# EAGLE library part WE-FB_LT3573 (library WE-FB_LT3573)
Flyback Converter WE-FB for LT3573 - Input voltage: 24 V - Output power: 5 W - Isolation voltage: 1.5 kV - designd for LT3573 -- Industrial input voltage
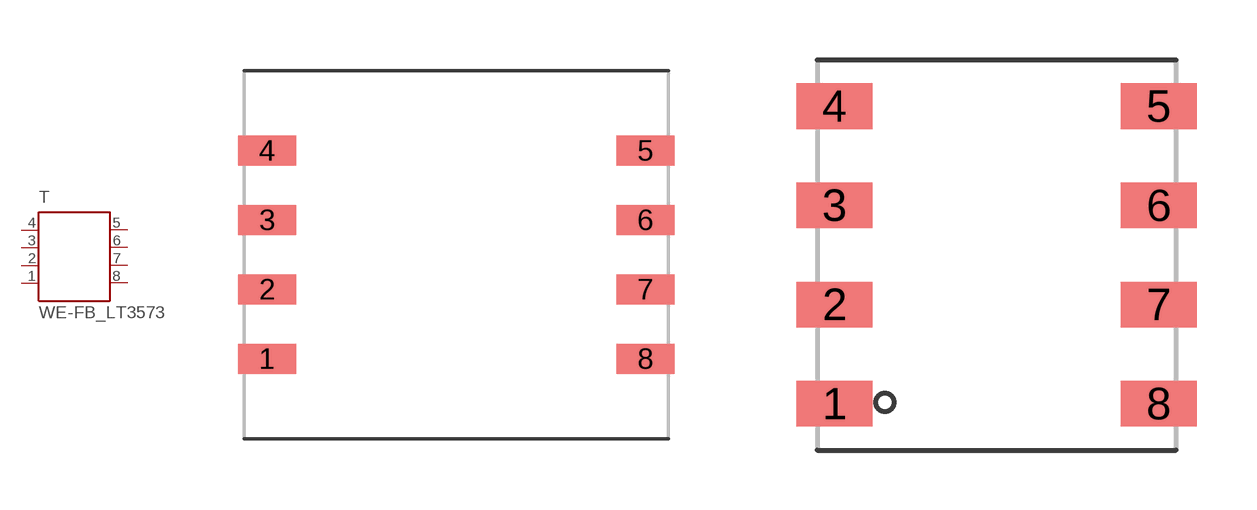
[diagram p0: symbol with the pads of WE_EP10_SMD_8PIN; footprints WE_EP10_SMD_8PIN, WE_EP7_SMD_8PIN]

Designator prefix T

## WE-FB_LT3573-750310471_WE-FB_EP10 (MPN: 750310471; OC_FARNELL: 1748681; OC_NEWARK: 34R6109; PACKAGE: EP10; SUPPLIER: Würth Elektronik eiSos GmbH), WE-FB_LT3573-750310559_WE-FB_EP10 (MPN: 750310559; OC_FARNELL: 1748680; OC_NEWARK: 34R6110; PACKAGE: EP10; SUPPLIER: Würth Elektronik eiSos GmbH), WE-FB_LT3573-750310562_WE-FB_EP10 (MPN: 750310562; OC_FARNELL: 1748682; OC_NEWARK: 34R6111; PACKAGE: EP10; SUPPLIER: Würth Elektronik eiSos GmbH), WE-FB_LT3573-750310563_WE-FB_EP10 (MPN: 750310563; OC_FARNELL: 1748685; OC_NEWARK: 34R6112; PACKAGE: EP10; SUPPLIER: Würth Elektronik eiSos GmbH), WE-FB_LT3573-750310564_WE-FB_EP10 (MPN: 750310564; OC_FARNELL: 1748686; OC_NEWARK: 34R6113; PACKAGE: EP10; SUPPLIER: Würth Elektronik eiSos GmbH), WE-FB_LT3573-750311303_WE-FB_EP10 (MPN: 750311303; OC_FARNELL: 1895732; OC_NEWARK: 47T5821; PACKAGE: EP10; SUPPLIER: Würth Elektronik eiSos GmbH), WE-FB_LT3573-750311304_WE-FB_EP10 (MPN: 750311304; OC_FARNELL: 1895733; OC_NEWARK: 47T5822; PACKAGE: EP10; SUPPLIER: Würth Elektronik eiSos GmbH), WE-FB_LT3573-750311305_WE-FB_EP10 (MPN: 750311305; OC_FARNELL: 1895735; OC_NEWARK: 47T5823; PACKAGE: EP10; SUPPLIER: Würth Elektronik eiSos GmbH), WE-FB_LT3573-750311306_WE-FB_EP10 (MPN: 750311306; OC_FARNELL: 1895736; OC_NEWARK: 47T5824; PACKAGE: EP10; SUPPLIER: Würth Elektronik eiSos GmbH), WE-FB_LT3573-750311307_WE-FB_EP10 (MPN: 750311307; OC_FARNELL: 1895737; OC_NEWARK: 47T5825; PACKAGE: EP10; SUPPLIER: Würth Elektronik eiSos GmbH), WE-FB_LT3573-750311308_WE-FB_EP10 (MPN: 750311308; OC_FARNELL: 1895738; OC_NEWARK: 47T5826; PACKAGE: EP10; SUPPLIER: Würth Elektronik eiSos GmbH), WE-FB_LT3573-750311567_WE-FB_EP10 (MPN: 750311567; OC_FARNELL: 1895740; OC_NEWARK: 47T5839; PACKAGE: EP10; SUPPLIER: Würth Elektronik eiSos GmbH), WE-FB_LT3573-750311675_WE-FB_EP10 (MPN: 750311675; OC_FARNELL: 1895739; OC_NEWARK: 47T5858; PACKAGE: EP10; SUPPLIER: Würth Elektronik eiSos GmbH)  [WE_EP10_SMD_8PIN]
1  1  pas
2  2  pas
3  3  pas
4  4  pas
5  5  pas
6  6  pas
7  7  pas
8  8  pas

## WE-FB_LT3573-750310799_WE-FB_EP7 (MPN: 750310799; OC_FARNELL: 1748689; OC_NEWARK: 34R6114; PACKAGE: EP7_SMD_8PIN; SUPPLIER: Würth Elektronik eiSos GmbH), WE-FB_LT3573-750311692_WE-FB_EP7 (MPN: 750311692; OC_FARNELL: 1895728; OC_NEWARK: 47T5862; PACKAGE: EP7_SMD_8PIN; SUPPLIER: Würth Elektronik eiSos GmbH), WE-FB_LT3573-750370040_WE-FB_EP7 (MPN: 750370040; OC_FARNELL: 1748687; OC_NEWARK: 34R6115; PACKAGE: EP7_SMD_8PIN; SUPPLIER: Würth Elektronik eiSos GmbH), WE-FB_LT3573-750370041_WE-FB_EP7 (MPN: 750370041; OC_FARNELL: 1748688; OC_NEWARK: 34R6116; PACKAGE: EP7_SMD_8PIN; SUPPLIER: Würth Elektronik eiSos GmbH)  [WE_EP7_SMD_8PIN]
Pads as for WE_EP10_SMD_8PIN

## WE-FB_LT3573-750370047_WE-FB_750370047 (MPN: 750370047; OC_FARNELL: 1748690; OC_NEWARK: 34R6118; PACKAGE: EP7; SUPPLIER: Würth Elektronik eiSos GmbH)  [WE_EP7*_750370047]
Pads as for WE_EP10_SMD_8PIN

## WE-FB_LT3573_WE-FB_750370058_750370059  [WE_EP7*_750370058_750370059]
Pads as for WE_EP10_SMD_8PIN

## WE-FB_LT3573-750370042_WE-FB_ER9.5 (MPN: 750370042; OC_FARNELL: 1748691; OC_NEWARK: 34R6117; PACKAGE: ER9.5; SUPPLIER: Würth Elektronik eiSos GmbH)  [WE_ER9.5_SMD_8PIN]
1  4  pas
2  3  pas
3  2  pas
4  1  pas
5  8  pas
6  7  pas
7  6  pas
8  5  pas

## Footprint WE_EP10_SMD_8PIN (pad centres in mm)
Transformer, EP10 SMD 8 Pin
smd 2.08 x 1.07: 1 -6.78,-3.735; 2 -6.78,-1.245; 3 -6.78,1.245; 4 -6.78,3.735; 5 6.78,3.735; 6 6.78,1.245; 7 6.78,-1.245; 8 6.78,-3.735

## Footprint WE_EP7_SMD_8PIN (pad centres in mm)
Transformer, EP7 SMD 8 Pin
smd 1.91 x 1.143: 1 -4.065,-3.735; 2 -4.065,-1.245; 3 -4.065,1.245; 4 -4.065,3.735; 5 4.065,3.735; 6 4.065,1.245; 7 4.065,-1.245; 8 4.065,-3.735

## Footprint WE_EP7*_750370047 (pad centres in mm)
Transformer, EP7* SMD 8Pin für WE-FB
smd 1.96 x 1.17: 1 -6.16,-3.735; 2 -6.16,-1.245; 3 -6.16,1.245; 4 -6.16,3.735; 5 6.16,3.735; 6 6.16,1.245; 7 6.16,-1.245; 8 6.16,-3.735

## Footprint WE_EP7*_750370058_750370059 (pad centres in mm)
Transformer, EP7* SMD 8Pin für WE-FB
smd 1.96 x 1.17: 1 -5.83,-3.75; 2 -5.83,-1.25; 3 -5.83,1.25; 4 -5.83,3.75; 5 5.83,3.75; 6 5.83,1.25; 7 5.83,-1.25; 8 5.83,-3.75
